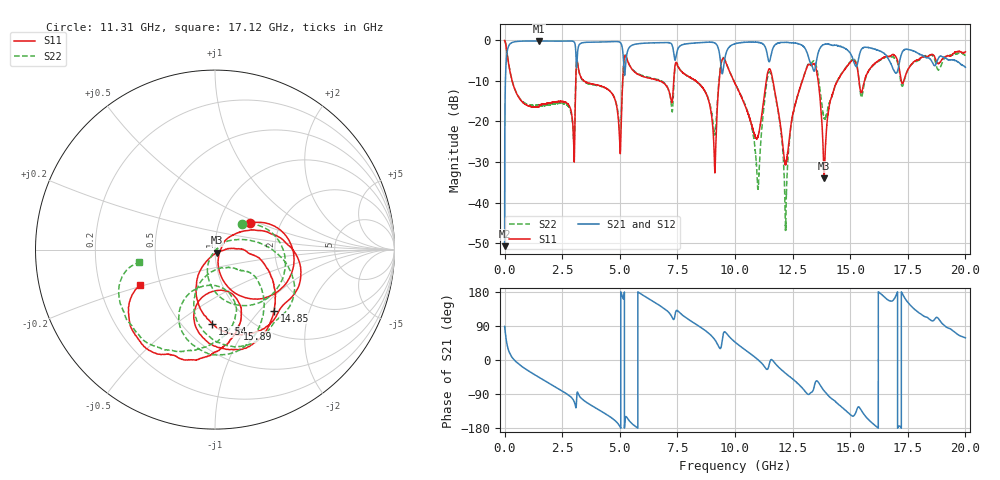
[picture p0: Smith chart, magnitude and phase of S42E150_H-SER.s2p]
!{S42E150}
!Johanson Technology Inc.
!www.johansontechnology.com
!Test Board Conditions:
!Substrate Type  RO4350B
!Substrate Thickness  50 mil
!Substrate Dk  3.66
!TL Type: GCPW
!TL Trace Width  60 mil
!TL Gap  10 mil
!Electrode orientation  Horizontal
!DUT TOPOLOGY	SERIES
!Mounting Pad LxW  14x55 mil
! Created Wed Nov 25 21:59:39 2020
# khz S ma R 50
! 2 Port Network Data from SP1.SP block
! freq  magS11  angS11  magS21  angS21  magS12  angS12  magS22  angS22
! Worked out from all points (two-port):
!   20001 points, 300 kHz to 20 GHz, reference 50 ohm
!   highest |S21| = -0.13 dB at 1.506 GHz (marker M1); lowest = -50.8 dB at 300 kHz (marker M2)
!   |S21| within 3 dB of the highest: 102.2 MHz to 3.093 GHz (2.99 GHz wide, 187 % of centre); 5.314 GHz to 7.343 GHz (2.029 GHz wide, 32.1 % of centre)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
!   lowest |S11| = -34.0 dB at 13.87 GHz (marker M3), VSWR 1.04, Z = 50.9 - j1.8 ohm
!   |S11| at or under -10 dB: 327 MHz to 3.089 GHz (2.762 GHz wide, 162 % of centre); 3.449 GHz to 5.126 GHz (1.677 GHz wide, 39.1 % of centre); 9.95 GHz to 11.36 GHz (1.407 GHz wide, 13.2 % of centre)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
!   |S22| runs from -46.9 to 0.0 dB; largest |S21 - S12| = 0.017
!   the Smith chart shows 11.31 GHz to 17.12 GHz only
!   S11 on the Smith chart (normalised r, x): 11.31 GHz: 1.41, +0.44; 13.54 GHz: 0.69, -0.69; 14.85 GHz: 1.37, -1.20; 15.89 GHz: 0.82, -0.92; 17.12 GHz: 0.39, -0.19
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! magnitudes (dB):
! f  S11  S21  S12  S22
! 300 kHz  0.0  -50.8  -50.7  0.0
! 175.3 MHz  -5.8  -1.4  -1.4  -5.7
! 1.506 GHz  -15.9  -0.1  -0.1  -16.2
! 3.334 GHz  -9.3  -0.6  -0.6  -9.4
! 4.98 GHz  -23.2  -0.4  -0.4  -21.4
! 5.258 GHz  -3.8  -5.6  -5.5  -3.8
! 6.667 GHz  -9.8  -0.6  -0.6  -9.7
! 9.105 GHz  -29.4  -0.6  -0.6  -22.9
! 9.445 GHz  -4.7  -8.2  -8.2  -4.4
! 10 GHz  -10.6  -0.8  -0.8  -10.5
! 10.99 GHz  -23.9  -0.5  -0.5  -36.3
! 11.31 GHz  -12.2  -1.5  -1.5  -13.7
! 11.63 GHz  -9.3  -2.3  -2.3  -9.8
! 12.2 GHz  -30.6  -0.5  -0.4  -45.1
! 13.33 GHz  -6.2  -6.1  -6.1  -5.5
! 13.54 GHz  -7.7  -4.8  -4.9  -6.6
! 13.87 GHz  -34.0  -1.0  -1.0  -19.1
! 14.85 GHz  -6.5  -2.2  -2.2  -6.4
! 15.89 GHz  -6.8  -1.9  -1.8  -6.8
! 16.67 GHz  -4.0  -4.6  -4.8  -3.8
! 17.12 GHz  -6.8  -5.8  -5.9  -7.5
! 20 GHz  -2.8  -6.6  -6.6  -3.8
